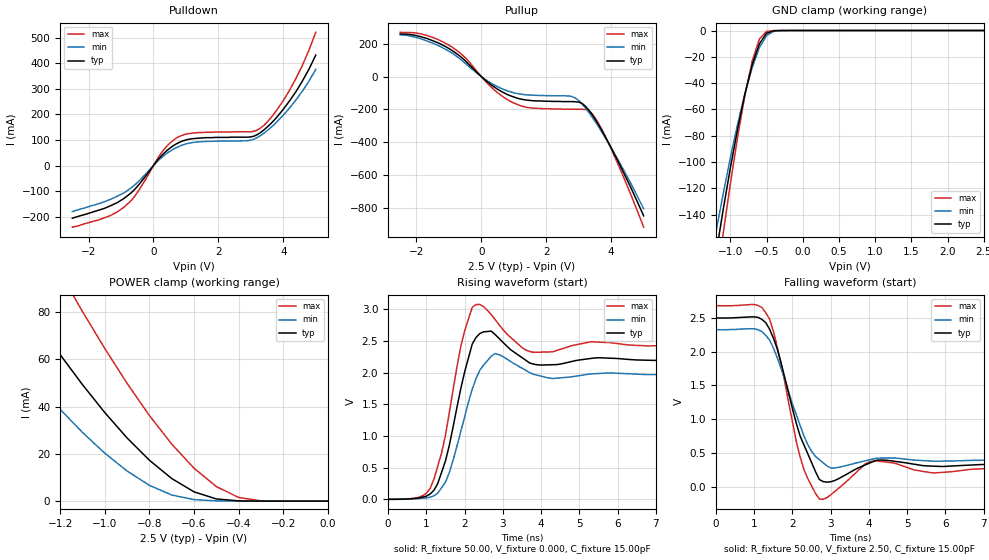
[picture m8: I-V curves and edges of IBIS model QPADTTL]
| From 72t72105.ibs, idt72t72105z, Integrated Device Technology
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|   Model QPADTTL
[Model]   QPADTTL
Model_type   3-state
Polarity   Non-Inverting
Enable   Active-High
Vmeas =  1.250V
C_comp   3.00pF   NA   NA
[Temperature Range]   25.00   85.00   -40.00
[Voltage Range]   2.50V   2.30V   2.70V
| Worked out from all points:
|   slope of the pulldown table from 0 to 0.375 V, typ, clamps not added: 6.94 ohm
|   slope of the pullup table from 0 to 0.375 V, typ, clamps not added: 6.23 ohm
|   GND clamp passes 1 mA (typ) near -0.45 V on its own axis
|   POWER clamp passes 1 mA (typ) near -0.50 V on its own axis
|   rising waveform, R_fixture 50.00, V_fixture 0.000, C_fixture 15.00pF: 20-80 % time 499ps typ, 540ps min, 481ps max; typ from 0 V to 2.2 V
|   falling waveform, R_fixture 50.00, V_fixture 2.50, C_fixture 15.00pF: 20-80 % time 608ps typ, 700ps min, 529ps max; typ from 2.5 V to 0.321 V
[Pulldown]
| voltage   I(typ)   I(min)   I(max)
-2.5V     -206mA     -180mA     -241mA
-1.5V     -167mA     -141mA     -204mA
-900mV    -128mA     -106mA     -162mA
-500mV    -82.28mA   -67.22mA   -106mA
300mV     45.13mA    36.58mA    59.01mA
800mV     90.82mA    75.57mA    114mA
1.4V      107mA      92.58mA    129mA
3V        112mA      99.27mA    132mA
3.4V      139mA      126mA      157mA
4.2V      254mA      226mA      296mA
4.6V      333mA      293mA      395mA
5V        432mA      376mA      521mA
[Pullup]
| voltage   I(typ)   I(min)   I(max)
-2.5V     260mA      255mA      270mA
-1.7V     234mA      219mA      252mA
-900mV    159mA      143mA      180mA
-500mV    97.12mA    81.41mA    116mA
200mV     -34.29mA   -27.66mA   -43.74mA
1V        -124mA     -98.21mA   -161mA
1.5V      -145mA     -112mA     -190mA
2.8V      -152mA     -122mA     -199mA
3.1V      -163mA     -166mA     -199mA
3.3V      -202mA     -215mA     -206mA
3.8V      -360mA     -367mA     -356mA
5V        -848mA     -805mA     -917mA
[GND_clamp]
| voltage   I(typ)   I(min)   I(max)
-2.5V     -663mA     -589mA     -765mA
-1.2V     -170mA     -153mA     -195mA
-1.1V     -136mA     -124mA     -154mA
-1V       -104mA     -96.2mA    -116mA
-900mV    -74.56mA   -70.77mA   -80.61mA
-800mV    -48.24mA   -47.87mA   -49.04mA
-700mV    -26.16mA   -28.23mA   -23.28mA
-600mV    -10.07mA   -12.98mA   -6.406mA
-500mV    -2.002mA   -3.724mA   -655uA
-400mV    -177uA     -538uA     -28.12uA
-300mV    -7.848uA   -44.31uA   -410nA
2.5V      25.16nA    97.83nA    24.47nA
[POWER_clamp]
| voltage   I(typ)   I(min)   I(max)
-2.5V     256mA      206mA      321mA
-1.6V     118mA      84.74mA    166mA
-1.4V     89.24mA    60.62mA    131mA
-1.3V     75.3mA     49.37mA    113mA
-1.2V     61.92mA    38.79mA    96.5mA
-1.1V     49.24mA    29.04mA    80.16mA
-800mV    17.3mA     6.679mA    36.2mA
-600mV    3.925mA    651uA      13.91mA
-500mV    924uA      114uA      6.162mA
-400mV    104uA      14.03uA    1.537mA
-300mV    6.378uA    1.193uA    142uA
0V        25.16nA    29.25nA    27nA
[Ramp]
| variable   typ   min   max
dV/dt_r   1.34/0.36n   1.20/0.43n   1.48/0.31n
dV/dt_f   1.33/0.51n   1.18/0.59n   1.48/0.44n
R_load = 50.00
[Rising Waveform]
R_fixture = 50.00
V_fixture = 0.000
C_fixture = 15.00pF
R_dut = 0.75
L_dut = 8.10nH
C_dut = 0.53pF
| time   V(typ)   V(min)   V(max)
0s        0V         0V         0V
1.1ns     84.43mV    33.72mV    172mV
1.4ns     428mV      184mV      736mV
1.6ns     850mV      421mV      1.366V
2ns       2.008V     1.299V     2.656V
2.3ns     2.556V     1.907V     3.076V
2.8ns     2.601V     2.301V     2.837V
3.8ns     2.135V     1.974V     2.321V
5.3ns     2.224V     1.979V     2.488V
9.9ns     2.202V     1.973V     2.436V
[Falling Waveform]
R_fixture = 50.00
V_fixture = 2.50
C_fixture = 15.00pF
R_dut = 0.75
L_dut = 8.10nH
C_dut = 0.53pF
| time   V(typ)   V(min)   V(max)
0s        2.5V       2.325V     2.681V
1.1ns     2.508V     2.325V     2.685V
1.4ns     2.335V     2.174V     2.483V
1.6ns     2.044V     1.912V     2.071V
2.2ns     748mV      906mV      439mV
2.7ns     106mV      400mV      -183mV
3.1ns     88.98mV    276mV      -75.49mV
4.1ns     369mV      408mV      377mV
5.7ns     302mV      376mV      202mV
9.9ns     321mV      388mV      254mV
